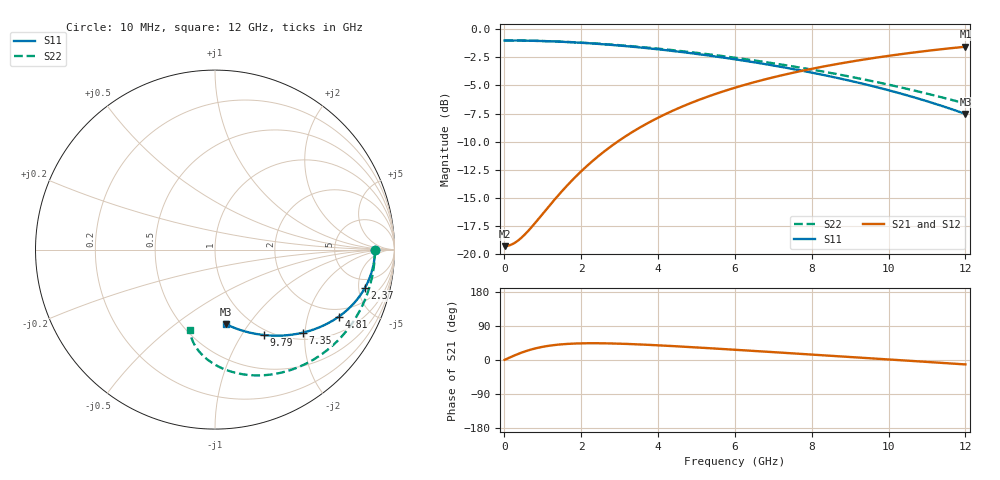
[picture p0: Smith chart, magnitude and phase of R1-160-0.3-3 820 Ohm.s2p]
!version-1
!date-03.2021
# MHz S RI R 50
!Freq ReS11 ImS11 ReS21 ImS21 ReS12 ImS12 ReS22 ImS22
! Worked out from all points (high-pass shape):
!   601 points, 10 MHz to 12 GHz, reference 50 ohm
!   highest |S21| = -1.56 dB at 12 GHz (marker M1); lowest = -19.3 dB at 10 MHz (marker M2)
!   |S21| within 3 dB of the highest: 6.672 GHz to end of sweep
!   lowest |S11| = -7.5 dB at 12 GHz (marker M3), VSWR 2.45, Z = 39 - j39.4 ohm
!   |S11| at or under -10 dB: nowhere
!   |S22| runs from -6.6 to -1.0 dB; largest |S21 - S12| = 0
!   S11 on the Smith chart (normalised r, x): 10 MHz: 17, -0; 2.37 GHz: 3.55, -5.89; 4.81 GHz: 1.63, -3.17; 7.35 GHz: 1.15, -1.95; 9.79 GHz: 0.92, -1.26; 12 GHz: 0.78, -0.79
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10  0.8913 -0.000946  0.1087 0.000881  0.1087 0.000881  0.8913 -0.00201
250  0.8907 -0.0236  0.1097 0.022  0.1097 0.022  0.8896 -0.0501
510  0.8886 -0.0481  0.1128 0.0447  0.1128 0.0447  0.8841 -0.1019
1230  0.8758 -0.1147  0.1319 0.105  0.1319 0.105  0.8505 -0.2406
1630  0.8643 -0.1503  0.1489 0.1358  0.1489 0.1358  0.8208 -0.3126
2010  0.8508 -0.1829  0.1687 0.1627  0.1687 0.1627  0.7862 -0.3766
2370  0.8357 -0.2126  0.1905 0.1857  0.1905 0.1857  0.7484 -0.4325
2790  0.8157 -0.2454  0.2191 0.209  0.2191 0.209  0.6992 -0.4914
3190  0.7943 -0.2748  0.249 0.2275  0.249 0.2275  0.6483 -0.5407
3590  0.7709 -0.3022  0.2809 0.2421  0.2809 0.2421  0.5944 -0.5831
4010  0.7446 -0.3288  0.316 0.2534  0.316 0.2534  0.5358 -0.6203
4810  0.6899 -0.3734  0.3855 0.2629  0.3855 0.2629  0.4223 -0.6705
5390  0.6472 -0.4006  0.4365 0.2605  0.4365 0.2605  0.3414 -0.6913
6010  0.5993 -0.4252  0.4902 0.2497  0.4902 0.2497  0.2589 -0.7006
6650  0.5478 -0.4457  0.5436 0.2304  0.5436 0.2304  0.1797 -0.6979
7350  0.4893 -0.4627  0.5987 0.2006  0.5987 0.2006  0.1018 -0.6833
8010  0.4323 -0.4734  0.6467 0.1649  0.6467 0.1649  0.0379 -0.6604
8910  0.3519 -0.4797  0.7046 0.1058  0.7046 0.1058  -0.0336 -0.619
9790  0.2708 -0.4758  0.7516 0.0375  0.7516 0.0375  -0.0853 -0.5713
10010  0.2501 -0.4732  0.7617 0.019  0.7617 0.019  -0.0955 -0.5587
10990  0.1572 -0.4529  0.7979 -0.0695  0.7979 -0.0695  -0.1274 -0.5021
12000  0.0612 -0.416  0.8185 -0.1693  0.8185 -0.1693  -0.1388 -0.4467
